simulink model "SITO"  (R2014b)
settings: Solver=ode5  SolverMode=SingleTasking  StartTime=0.0  StopTime=60  FixedStep=0.001  RelTol=1e-3
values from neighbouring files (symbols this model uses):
  a_poz = conv([1 0],[T_poz 1])    [SITOrizeniP.m]    (also in SITOrizeniPD.m)
  a_uhel = conv([T1_uhel 1], [T2_uhel*T2_uhel, 2*ksi*T2_uhel, 1])    [SITOrizeniP.m]    (also in SITOrizeniPD.m)
  b_poz = [k_poz]    [SITOrizeniP.m]    (also in SITOrizeniPD.m)
  b_uhel = [k_uhel, 0]    [SITOrizeniP.m]    (also in SITOrizeniPD.m)
  p_poz = [1 p0_poz]    [SITOrizeniP.m]    (also in SITOrizeniPD.m)
  p_uhel = [1]    [SITOrizeniP.m]    (also in SITOrizeniPD.m = [alfa*Td, 1])
  q_poz = [D_poz P_poz]    [SITOrizeniP.m]    (also in SITOrizeniPD.m)
  q_uhel = [Kp]    [SITOrizeniP.m]    (also in SITOrizeniPD.m = [Td*Kp*(alfa+1), Kp])
  r_poz = [R_poz]    [SITOrizeniP.m]    (also in SITOrizeniPD.m)
libraries: simulink x1

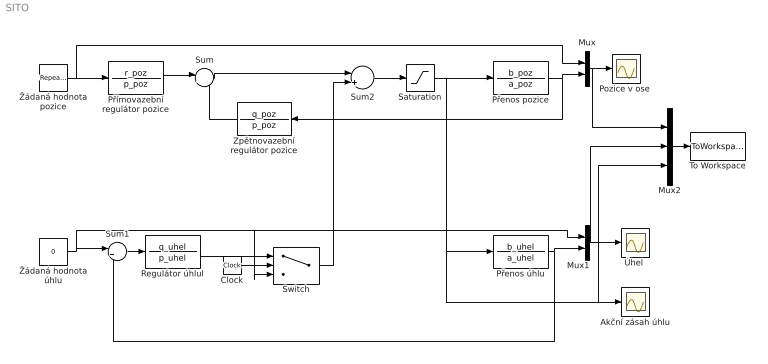
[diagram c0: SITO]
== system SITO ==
  Akční zásah úhlu : Scope
  Clock : Clock
  Mux : Mux  Inputs=2
  Mux1 : Mux  Inputs=2
  Mux2 : Mux  Inputs=3
  "Pozice v ose " : Scope
  Přenos pozice : TransferFcn  Numerator=b_poz  Denominator=a_poz
  Přenos úhlu : TransferFcn  Numerator=b_uhel  Denominator=a_uhel
  Přímovazební regulátor pozice : TransferFcn  Numerator=r_poz  Denominator=p_poz
  Regulátor úhlul : TransferFcn  Numerator=q_uhel  Denominator=p_uhel
  Saturation : Saturate  UpperLimit=1  LowerLimit=-1
  Sum : Sum  Inputs=|+-
  Sum1 : Sum  Inputs=|+-
  Sum2 : Sum  Inputs=|++
  Switch : Switch  Threshold=30
  To Workspace : ToWorkspace  VariableName=SITOreg  SaveFormat=Timeseries  SampleTime=-1
  Zpětnovazební regulátor pozice : TransferFcn  Numerator=q_poz  Denominator=p_poz
  "Úhel " : Scope
  Žádaná hodnota úhlu : Constant  Value=0
  Žádaná hodnota pozice : simulink/Sources/Repeating Sequence  rep_seq_t=[0 6 6.01 12 12.01 30]  rep_seq_y=[0.2 0.2 0.4 0.4 0.2 0.2]
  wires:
  Žádaná hodnota úhlu/1 -> Sum1/1, Switch/3, Mux1/1
  Sum1/1 -> Regulátor úhlul/1
  Přenos pozice/1 -> Mux/2, Zpětnovazební regulátor pozice/1
  Přenos úhlu/1 -> Mux1/2, Sum1/2
  Sum/1 -> Sum2/1
  Sum2/1 -> Saturation/1
  Mux/1 -> Mux2/1, "Pozice v ose "/1
  Mux1/1 -> Mux2/2, "Úhel "/1
  Žádaná hodnota pozice/1 -> Mux/1, Přímovazební regulátor pozice/1
  Clock/1 -> Switch/2
  Regulátor úhlul/1 -> Switch/1
  Switch/1 -> Sum2/2
  Zpětnovazební regulátor pozice/1 -> Sum/2
  Přímovazební regulátor pozice/1 -> Sum/1
  Saturation/1 -> Přenos pozice/1, Přenos úhlu/1, Mux2/3, Akční zásah úhlu/1
  Mux2/1 -> To Workspace/1
